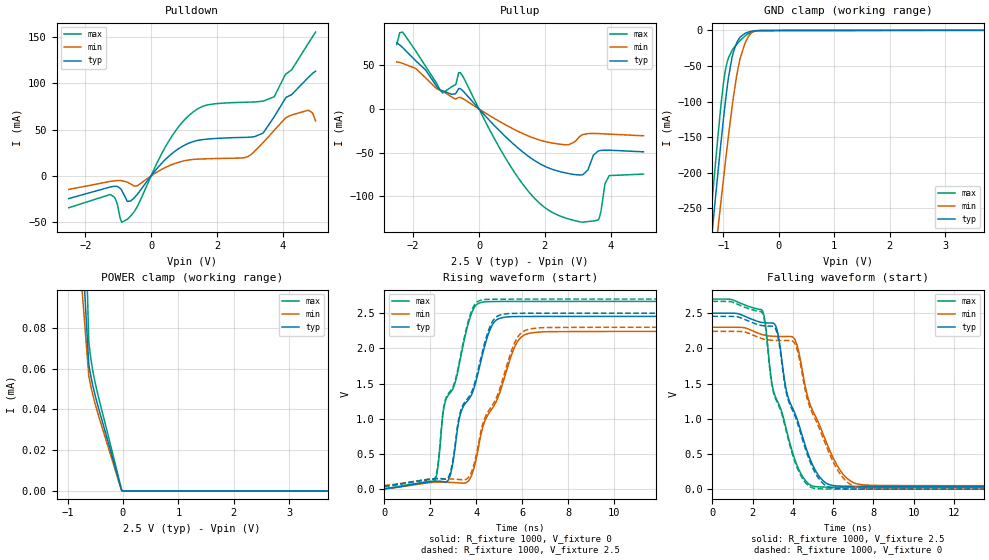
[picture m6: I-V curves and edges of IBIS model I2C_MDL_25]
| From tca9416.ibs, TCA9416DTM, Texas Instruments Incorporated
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[Model]   I2C_MDL_25
Model_type   I/O
Polarity   Non-Inverting
Enable   Active-High
Vinl = 0.75
Vinh = 1.75
Vmeas = 1.25
Vref = 0
Cref = 2pF
Rref = 100000
|   typ   min   max
C_comp   7.2608pF   6.6746pF   7.8469pF
[Voltage Range]   2.5   2.25   2.75
[Temperature Range]   27   125   -40
[Pullup Reference]   2.5   2.25   2.75
[Pulldown Reference]   0   0   0
[Power Clamp Reference]   2.5   2.25   2.75
[GND Clamp Reference]   0   0   0
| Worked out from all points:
|   slope of the pulldown table from 0 to 0.375 V, typ, clamps not added: 24.1 ohm
|   slope of the pullup table from 0 to 0.375 V, typ, clamps not added: 24.4 ohm
|   GND clamp passes 1 mA (typ) near -0.47 V on its own axis
|   POWER clamp passes 1 mA (typ) near -1.55 V on its own axis
|   rising waveform, R_fixture 1000, V_fixture 0: 20-80 % time 1.27ns typ, 1.41ns min, 1.08ns max; typ from 0.001 V to 2.46 V
|   falling waveform, R_fixture 1000, V_fixture 2.5: 20-80 % time 1.35ns typ, 1.54ns min, 1.24ns max; typ from 2.5 V to 0.039 V
|   rising waveform, R_fixture 1000, V_fixture 2.5: 20-80 % time 1.27ns typ, 1.41ns min, 1.08ns max; typ from 0.039 V to 2.5 V
|   falling waveform, R_fixture 1000, V_fixture 0: 20-80 % time 1.35ns typ, 1.54ns min, 1.23ns max; typ from 2.46 V to 0.001 V
[Pulldown]
|I2C_MDL_25
|   Voltage   I(typ)   I(min)   I(max)
-2.5V     -24.5mA    -14.66mA   -34.4mA
-1.24V    -11.97mA   -5.975mA   -20.19mA
-1.075V   -11.23mA   -5.229mA   -25.74mA
-887.5mV  -15.95mA   -5.156mA   -50.01mA
-722.5mV  -27.56mA   -6.759mA   -46.95mA
1.055V    33.83mA    16.58mA    62.01mA
1.685V    39.64mA    18.44mA    76.36mA
2.945V    41.69mA    20.82mA    79.62mA
3.402V    46.16mA    35.83mA    80.69mA
3.74V     63.69mA    49.09mA    85.39mA
4.775V    106.1mA    70.88mA    142.9mA
5V        113mA      59.41mA    155.3mA
[GND Clamp]
|I2C_MDL_25
|   Voltage   I(typ)   I(min)   I(max)
-2.5V     -1.359A    -1.286A    -1.452A
-1.308V   -368.1mA   -428.8mA   -333.6mA
-1.18V    -264.1mA   -336.6mA   -218.3mA
-1.12V    -216.1mA   -293.6mA   -166mA
-1.052V   -163.6mA   -245.7mA   -111.1mA
-977.5mV  -108.9mA   -193.8mA   -62.22mA
-917.5mV  -70.89mA   -153.7mA   -40.56mA
-842.5mV  -37.21mA   -106.9mA   -27.9mA
-737.5mV  -14.09mA   -53.67mA   -17.58mA
-602.5mV  -4.048mA   -16.73mA   -7.558mA
-340mV    -316.2uA   -338.2uA   -410.1uA
5V        0A         0A         0A
[Pullup]
|I2C_MDL_25
|   Voltage   I(typ)   I(min)   I(max)
-2.5V     75.81mA    53.97mA    73.97mA
-2.32V    70.38mA    52.27mA    88.16mA
-1.105V   20.72mA    20.39mA    18.42mA
-707.5mV  17.71mA    11.35mA    27.97mA
-565mV    23.14mA    13.14mA    41.41mA
1.055V    -40.45mA   -23.13mA   -71.31mA
2.263V    -69.61mA   -39.25mA   -119.2mA
3.155V    -75.44mA   -29.38mA   -129.8mA
3.62V     -48.24mA   -28.19mA   -127.3mA
3.83V     -47.16mA   -28.56mA   -85.58mA
3.958V    -47.22mA   -28.81mA   -76.37mA
5V        -49.14mA   -30.73mA   -74.59mA
[POWER Clamp]
|I2C_MDL_25
|   Voltage   I(typ)   I(min)   I(max)
-2.5V     145.3mA    82.03mA    233.2mA
-1.292V   387.8uA    292.4uA    747.9uA
-617.5mV  62.03uA    56.27uA    73.09uA
-595mV    58.44uA    53.19uA    67.98uA
-565mV    54.23uA    49.48uA    62.26uA
-535mV    50.51uA    46.11uA    57.52uA
-490mV    45.55uA    41.52uA    51.57uA
-32.5mV   1.007uA    661.4nA    1.448uA
-25mV     273.1nA    330.7nA    625.8nA
-17.5mV   136.6nA    0A         312.9nA
-10mV     0A         0A         0A
5V        0A         0A         0A
[Ramp]
|I2C_MDL_25
| variable   typ   min   max
dV/dt_r   1.47/1.28E-09   1.34/1.41E-09   1.60/1.09E-09
dV/dt_f   1.48/1.35E-09   1.35/1.55E-09   1.60/1.24E-09
R_load = 1000
[Rising Waveform]
|I2C_MDL_25
R_fixture =   1000
C_fixture =   0
L_fixture =   0
V_fixture =   0
V_fixture_min = 0
V_fixture_max = 0
|   Time   V(typ)   V(min)   V(max)
0s        953.7uV    1.052mV    796.5uV
2.205ns   112.7mV    99.85mV    129.5mV
2.557ns   107.3mV    99.52mV    1.101V
2.777ns   130mV      97.71mV    1.337V
3.305ns   1.069V     88.09mV    1.857V
3.701ns   1.292V     139.3mV    2.415V
4.537ns   2.219V     1.075V     2.664V
5.813ns   2.452V     2.109V     2.666V
7.221ns   2.453V     2.238V     2.667V
219.7ns   2.455V     2.242V     2.667V
[Falling Waveform]
|I2C_MDL_25
R_fixture =   1000
C_fixture =   0
L_fixture =   0
V_fixture =   2.5
V_fixture_min = 2.3
V_fixture_max = 2.7
|   Time   V(typ)   V(min)   V(max)
0s        2.5V       2.3V       2.7V
2.469ns   2.368V     2.196V     2.54V
3.129ns   2.329V     2.17V      1.316V
3.701ns   1.371V     2.169V     817.1mV
4.097ns   1.081V     2.124V     420.7mV
4.757ns   501.3mV    1.29V      81.86mV
5.329ns   173.7mV    904.7mV    32.59mV
6.605ns   42.71mV    176.4mV    28.59mV
8.321ns   39.87mV    53.32mV    28.05mV
219.7ns   39.26mV    50.04mV    27.8mV
[Rising Waveform]
|I2C_MDL_25
R_fixture =   1000
C_fixture =   0
L_fixture =   0
V_fixture =   2.5
V_fixture_min = 2.3
V_fixture_max = 2.7
|   Time   V(typ)   V(min)   V(max)
0s        39.26mV    50.04mV    27.8mV
2.205ns   151.3mV    148.9mV    157mV
2.557ns   145.4mV    148mV      1.125V
2.777ns   168mV      146.2mV    1.359V
3.305ns   1.102V     136.6mV    1.889V
3.701ns   1.325V     188.1mV    2.448V
4.493ns   2.224V     1.095V     2.696V
5.813ns   2.498V     2.169V     2.699V
7.177ns   2.499V     2.296V     2.7V
219.7ns   2.5V       2.3V       2.7V
[Falling Waveform]
|I2C_MDL_25
R_fixture =   1000
C_fixture =   0
L_fixture =   0
V_fixture =   0
V_fixture_min = 0
V_fixture_max = 0
|   Time   V(typ)   V(min)   V(max)
0s        2.455V     2.242V     2.667V
2.469ns   2.324V     2.138V     2.509V
3.129ns   2.285V     2.113V     1.292V
3.657ns   1.389V     2.111V     836.9mV
4.097ns   1.044V     2.066V     391mV
4.757ns   459.5mV    1.237V     54.23mV
5.329ns   134.6mV    849.8mV    5.543mV
6.605ns   4.373mV    125.6mV    1.58mV
8.321ns   1.563mV    4.27mV     1.046mV
219.7ns   953.8uV    1.052mV    796.6uV
